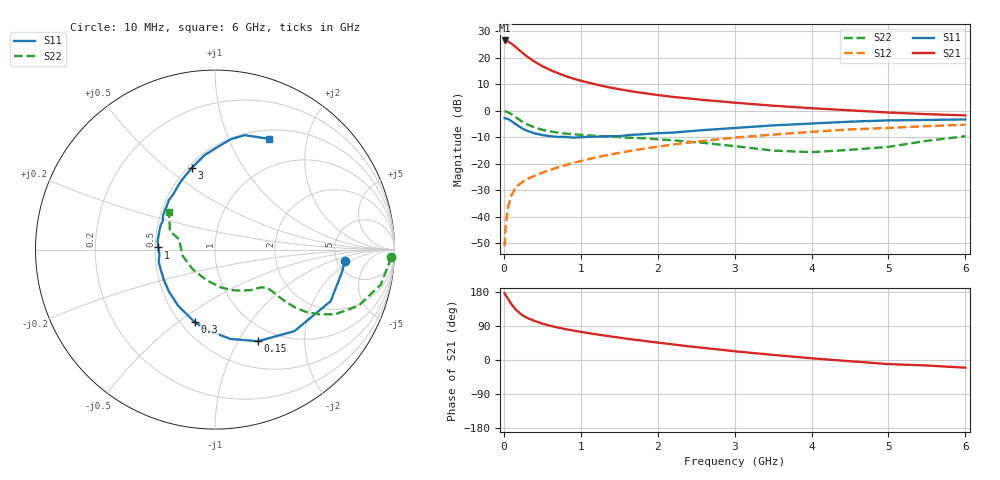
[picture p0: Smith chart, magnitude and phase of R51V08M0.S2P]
! SIEMENS Small Signal Semiconductors
! BFR183
! Si NPN RF Bipolar Junction Transistor in SOT23
! VCE = 1 V  IC = 8 mA
! Common Emitter S-Parameters:  May  1996
# GHz  S  MA  R  50
!  f  S11  S21  S12  S22
! GHz  MAG  ANG  MAG  ANG  MAG  ANG  MAG  ANG
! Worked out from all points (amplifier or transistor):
!   36 points, 10 MHz to 6 GHz, reference 50 ohm
!   highest |S21| = 26.5 dB at 10 MHz (marker M1)
!   |S21| within 3 dB of that: start of sweep to 174.4 MHz
!   unconditionally stable (mu >= 1): 787.7 MHz to 2.744 GHz
!   at 250 MHz: K = 0.57, MSG = 24.2 dB, |S12| = -26.7 dB
!   at 1.4 GHz: K = 1.07, MAG = 10.9 dB, |S12| = -16.4 dB
!   at 6 GHz: K = 0.93, MSG = 1.8 dB, |S12| = -5.3 dB
!   S11 on the Smith chart (normalised r, x): 10 MHz: 5.83, -1.62; 150 MHz: 0.81, -1.22; 300 MHz: 0.59, -0.58; 1 GHz: 0.52, +0.01; 3 GHz: 0.52, +0.61; 6 GHz: 0.61, +1.42
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0.01  0.7258 -5.2  21.14 176.5  0.0028 87.2  0.9795 -2.4
0.02  0.7193 -9.7  21.08 172.6  0.0057 81.8  0.971 -4.9
0.05  0.7057 -24.0  20.42 162.4  0.0142 77.7  0.9444 -11.9
0.1  0.6339 -45.8  18.46 147.1  0.0256 69.6  0.8585 -21.4
0.15  0.5642 -64.8  16.05 134.1  0.0347 63.8  0.7614 -28.2
0.2  0.5054 -80.1  13.9 124.9  0.0411 60.5  0.68 -32.0
0.25  0.4548 -93.9  12.08 117.1  0.0462 58.4  0.6103 -34.5
0.3  0.4206 -105.5  10.6 111.3  0.0513 57.6  0.5569 -35.8
0.4  0.3744 -123.2  8.429 103.1  0.0595 57.5  0.4855 -36.4
0.5  0.3484 -137.0  6.921 96.0  0.0679 58.3  0.4385 -36.4
0.6  0.331 -149.5  5.894 90.5  0.0767 59.4  0.4081 -36.1
0.7  0.3221 -159.6  5.136 85.7  0.0853 60.2  0.3874 -36.1
0.8  0.3209 -167.6  4.518 81.5  0.0945 60.3  0.3709 -36.2
1  0.3163 177.8  3.683 74.3  0.1127 60.9  0.3516 -36.9
1.1  0.3235 171.4  3.388 71.1  0.1224 60.7  0.3438 -38.0
1.6  0.3457 147.0  2.398 56.2  0.1708 58.6  0.3113 -44.2
2.2  0.3874 126.5  1.823 41.1  0.2306 53.7  0.278 -55.7
3  0.4732 105.9  1.419 23.1  0.311 44.7  0.2154 -80.0
3.5  0.5294 96.3  1.245 13.4  0.3558 38.1  0.1775 -104.8
4.5  0.6224 81.7  1.019 -3.2  0.4445 25.3  0.1835 -169.1
5.5  0.6705 69.2  0.862 -14.5  0.5138 13.3  0.2713 157.7
6  0.6856 64.0  0.817 -20.3  0.5452 5.6  0.3308 140.6
